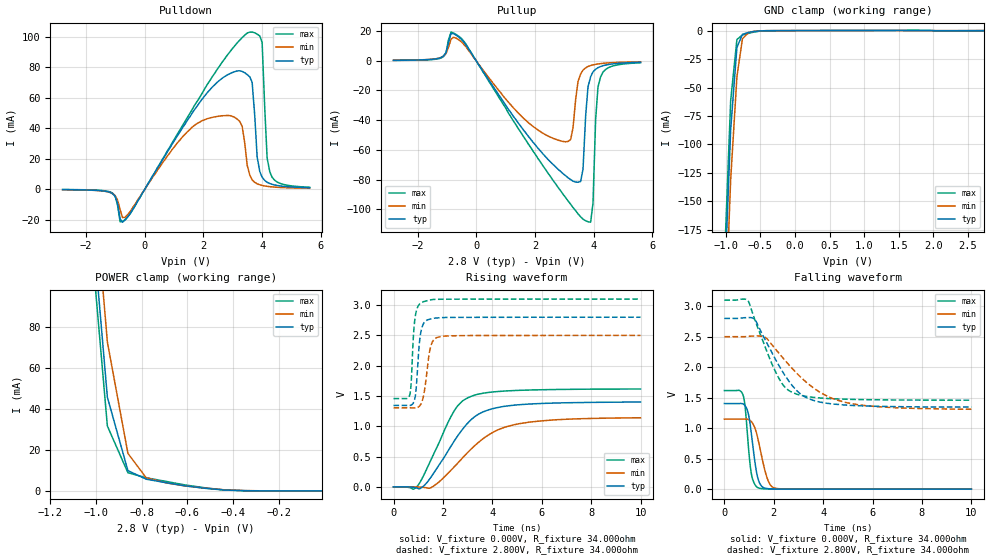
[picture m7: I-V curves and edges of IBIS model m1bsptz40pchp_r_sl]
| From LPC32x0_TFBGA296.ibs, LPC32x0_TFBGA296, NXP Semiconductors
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| |   Rev 0.20 IBIS Model Design Automation Generation   |
| |   N O N - S I L I C O N   C O R R E L A T E D   |
| |   This IBIS [Model] is pre-Beta tactical support   |
| |  Note: this IBIS [Model] contains clamp curves generated   |
| |   through simulation which should not be relied upon   |
| mem1bsptz40pchp
|   Bidirectional Pad 2.8
|   3state Output
|   Plain Input
|   1ns Slew Rate control
|   CMOS
| Repeater Mode (p1=1, p2=0)
[Model]   m1bsptz40pchp_r_sl | of mem1bsptz40pchp
Model_type   I/O
Polarity   Non-Inverting
Enable   Active-Low
|  Reciever Thresholds
Vinl   = 0.36V
Vinh   = 0.84V
| AC Test Load Conditions
Vref   = 0
Cref   = 1.2e-11
Rref   = 1000000000
Vmeas   = 0.6
| [Process Range]   typical   min   max
| C_comp edge width   400.000ps   400.000ps   400.000ps
| C_comp Tstrobe   40.000fs   40.000fs   40.000fs
C_comp   2.018pF   1.942pF   2.107pF
[Temperature Range]   25   125   -40
[Voltage Range]   2.80V   2.50V   3.10V
[GND Clamp Reference]   0.00V   0.00V   0.00V
[Pulldown Reference]   0.00V   0.00V   0.00V
[POWER Clamp Reference]   2.80V   2.50V   3.10V
[Pullup Reference]   2.80V   2.50V   3.10V
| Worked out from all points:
|   slope of the pulldown table from 0 to 0.42 V, typ, clamps not added: 31 ohm
|   slope of the pullup table from 0 to 0.42 V, typ, clamps not added: 32.9 ohm
|   GND clamp passes 1 mA (typ) near -0.61 V on its own axis
|   POWER clamp passes 1 mA (typ) near -0.49 V on its own axis
|   rising waveform, V_fixture 0.000V, R_fixture 34.000ohm: 20-80 % time 1.46ns typ, 1.87ns min, 1.14ns max; typ from 0 V to 1.4 V
|   falling waveform, V_fixture 0.000V, R_fixture 34.000ohm: 20-80 % time 280ps typ, 393ps min, 212ps max; typ from 1.4 V to 0 V
|   rising waveform, V_fixture 2.800V, R_fixture 34.000ohm: 20-80 % time 170ps typ, 240ps min, 143ps max; typ from 1.34 V to 2.8 V
|   falling waveform, V_fixture 2.800V, R_fixture 34.000ohm: 20-80 % time 1.31ns typ, 1.92ns min, 1.01ns max; typ from 2.8 V to 1.35 V
[GND Clamp]
| ref voltage   0.00V   0.00V   0.00V
|   Voltage   I(typ)   I(min)   I(max)
-2.8V     -3.643A    -3.653A    -3.644A
-1.01V    -211.8mA   -255.9mA   -186.6mA
-930mV    -86.6mA    -130.6mA   -61.24mA
-840mV    -14.83mA   -40.64mA   -7.829mA
-760mV    -3.203mA   -7.088mA   -3.83mA
-670mV    -1.622mA   -1.69mA    -2.382mA
-500mV    -233.9uA   -204.7uA   -414uA
2.73V     -11.67uA   31.94uA    -74.22uA
[Power Clamp]   | Vtable = Vcc - Vpad
| ref voltage   2.80V   2.50V   3.10V
|   Voltage   I(typ)   I(min)   I(max)
-2.82V    3.531A     3.518A     3.546A
-1.03V    149.7mA    178.4mA    134.4mA
-950mV    45.72mA    72.62mA    31.66mA
-860mV    9.875mA    18.31mA    8.866mA
-780mV    5.725mA    6.415mA    6.434mA
-690mV    3.961mA    3.875mA    4.58mA
-610mV    2.472mA    2.439mA    2.908mA
-440mV    442.3uA    569.4uA    500uA
-270mV    46.38uA    47.88uA    58.33uA
-10mV     1.584uA    1.118uA    2.104uA
[Pulldown]
| ref voltage   0.00V   0.00V   0.00V
|   Voltage   I(typ)   I(min)   I(max)
-2.8V     -319.3uA   -345.4uA   -253.1uA
-1.18V    -2.159mA   -2.186mA   -1.786mA
-670mV    -20.28mA   -18.52mA   -19.91mA
2.13V     63.32mA    46.22mA    68.69mA
3.24V     77.68mA    44.42mA    97.81mA
3.58V     73.7mA     9.097mA    103.1mA
3.66V     70.11mA    6.079mA    103.1mA
3.83V     21.16mA    3.502mA    101.8mA
4V        7.734mA    2.421mA    96.19mA
4.17V     4.509mA    1.835mA    20.55mA
4.26V     3.717mA    1.634mA    11.45mA
5.62V     949.5uA    582uA      1.271mA
[Pullup]   | Vtable = Vcc - Vpad
| ref voltage   2.80V   2.50V   3.10V
|   Voltage   I(typ)   I(min)   I(max)
-2.82V    285.4uA    305.9uA    228.1uA
-520mV    14.74mA    12.98mA    15.34mA
2.79V     -73.12mA   -53.48mA   -85.35mA
3.22V     -80.05mA   -52.98mA   -96.69mA
3.47V     -81.85mA   -13.92mA   -103.2mA
3.64V     -72.85mA   -6.25mA    -106.7mA
3.81V     -17.56mA   -3.872mA   -108.5mA
3.9V      -10.74mA   -3.234mA   -108.8mA
3.98V     -7.509mA   -2.77mA    -95.89mA
4.07V     -5.754mA   -2.418mA   -39.51mA
4.24V     -3.885mA   -1.924mA   -10.84mA
5.6V      -1.045mA   -712.7uA   -1.375mA
[Ramp]
R_load   = 34.000ohm
|   dV/dt(typ)   dV/dt(min)   dV/dt(max)
dV/dt_r   970.853mV/1.305ns   806.178mV/1.665ns   1.110V/1.040ns
dV/dt_f   1.001V/1.130ns   838.807mV/1.645ns   1.124V/890.000ps
[Rising Waveform]  | cubic spline decimation from 2001 points
V_fixture   = 0.000V
R_fixture   = 34.000ohm
|   Time   V(typ)   V(min)   V(max)
0s        4.292nV    139.7nV    2.459nV
810ps     -7.213mV   186uV      -37.6mV
975ps     -22.56mV   -1.932mV   16.58mV
1.21ns    11mV       -8.338mV   180.8mV
1.53ns    168.7mV    -10.11mV   458.1mV
2.46ns    757.9mV    331.6mV    1.257V
3.135ns   1.106V     621.6mV    1.493V
4.025ns   1.292V     900.5mV    1.567V
5.115ns   1.357V     1.045V     1.594V
10ns      1.4V       1.141V     1.615V
[Falling Waveform]  | cubic spline decimation from 2001 points
V_fixture   = 0.000V
R_fixture   = 34.000ohm
|   Time   V(typ)   V(min)   V(max)
0s        1.404V     1.148V     1.617V
750ps     1.398V     1.148V     1.55V
845ps     1.364V     1.149V     1.332V
970ps     1.236V     1.142V     712.1mV
1.08ns    952.4mV    1.112V     283.2mV
1.255ns   394.5mV    980.3mV    63.73mV
1.37ns    160.7mV    804.4mV    21.35mV
1.725ns   10.03mV    190.1mV    3.983mV
2.055ns   3.301mV    15.88mV    1.935mV
10ns      7.57uV     574.7uV    6.866uV
[Rising Waveform]  | cubic spline decimation from 2001 points
V_fixture   = 2.800V
V_fixture_min = 2.500V
V_fixture_max = 3.100V
R_fixture   = 34.000ohm
|   Time   V(typ)   V(min)   V(max)
0s        1.344V     1.305V     1.458V
660ps     1.344V     1.305V     1.522V
720ps     1.351V     1.304V     1.753V
825ps     1.402V     1.303V     2.6V
910ps     1.594V     1.304V     2.878V
1.065ns   2.438V     1.339V     3.022V
1.19ns    2.674V     1.457V     3.052V
1.465ns   2.767V     2.244V     3.084V
1.75ns    2.788V     2.464V     3.096V
10ns      2.8V       2.5V       3.1V
[Falling Waveform]  | cubic spline decimation from 2001 points
V_fixture   = 2.800V
V_fixture_min = 2.500V
V_fixture_max = 3.100V
R_fixture   = 34.000ohm
|   Time   V(typ)   V(min)   V(max)
0s        2.8V       2.5V       3.1V
965ps     2.814V     2.505V     3.084V
1.27ns    2.76V      2.512V     2.738V
1.67ns    2.434V     2.483V     2.312V
2.105ns   2.101V     2.279V     1.897V
2.42ns    1.885V     2.129V     1.687V
2.78ns    1.683V     1.964V     1.581V
3.525ns   1.466V     1.685V     1.509V
4.905ns   1.379V     1.422V     1.475V
10ns      1.346V     1.31V      1.459V
